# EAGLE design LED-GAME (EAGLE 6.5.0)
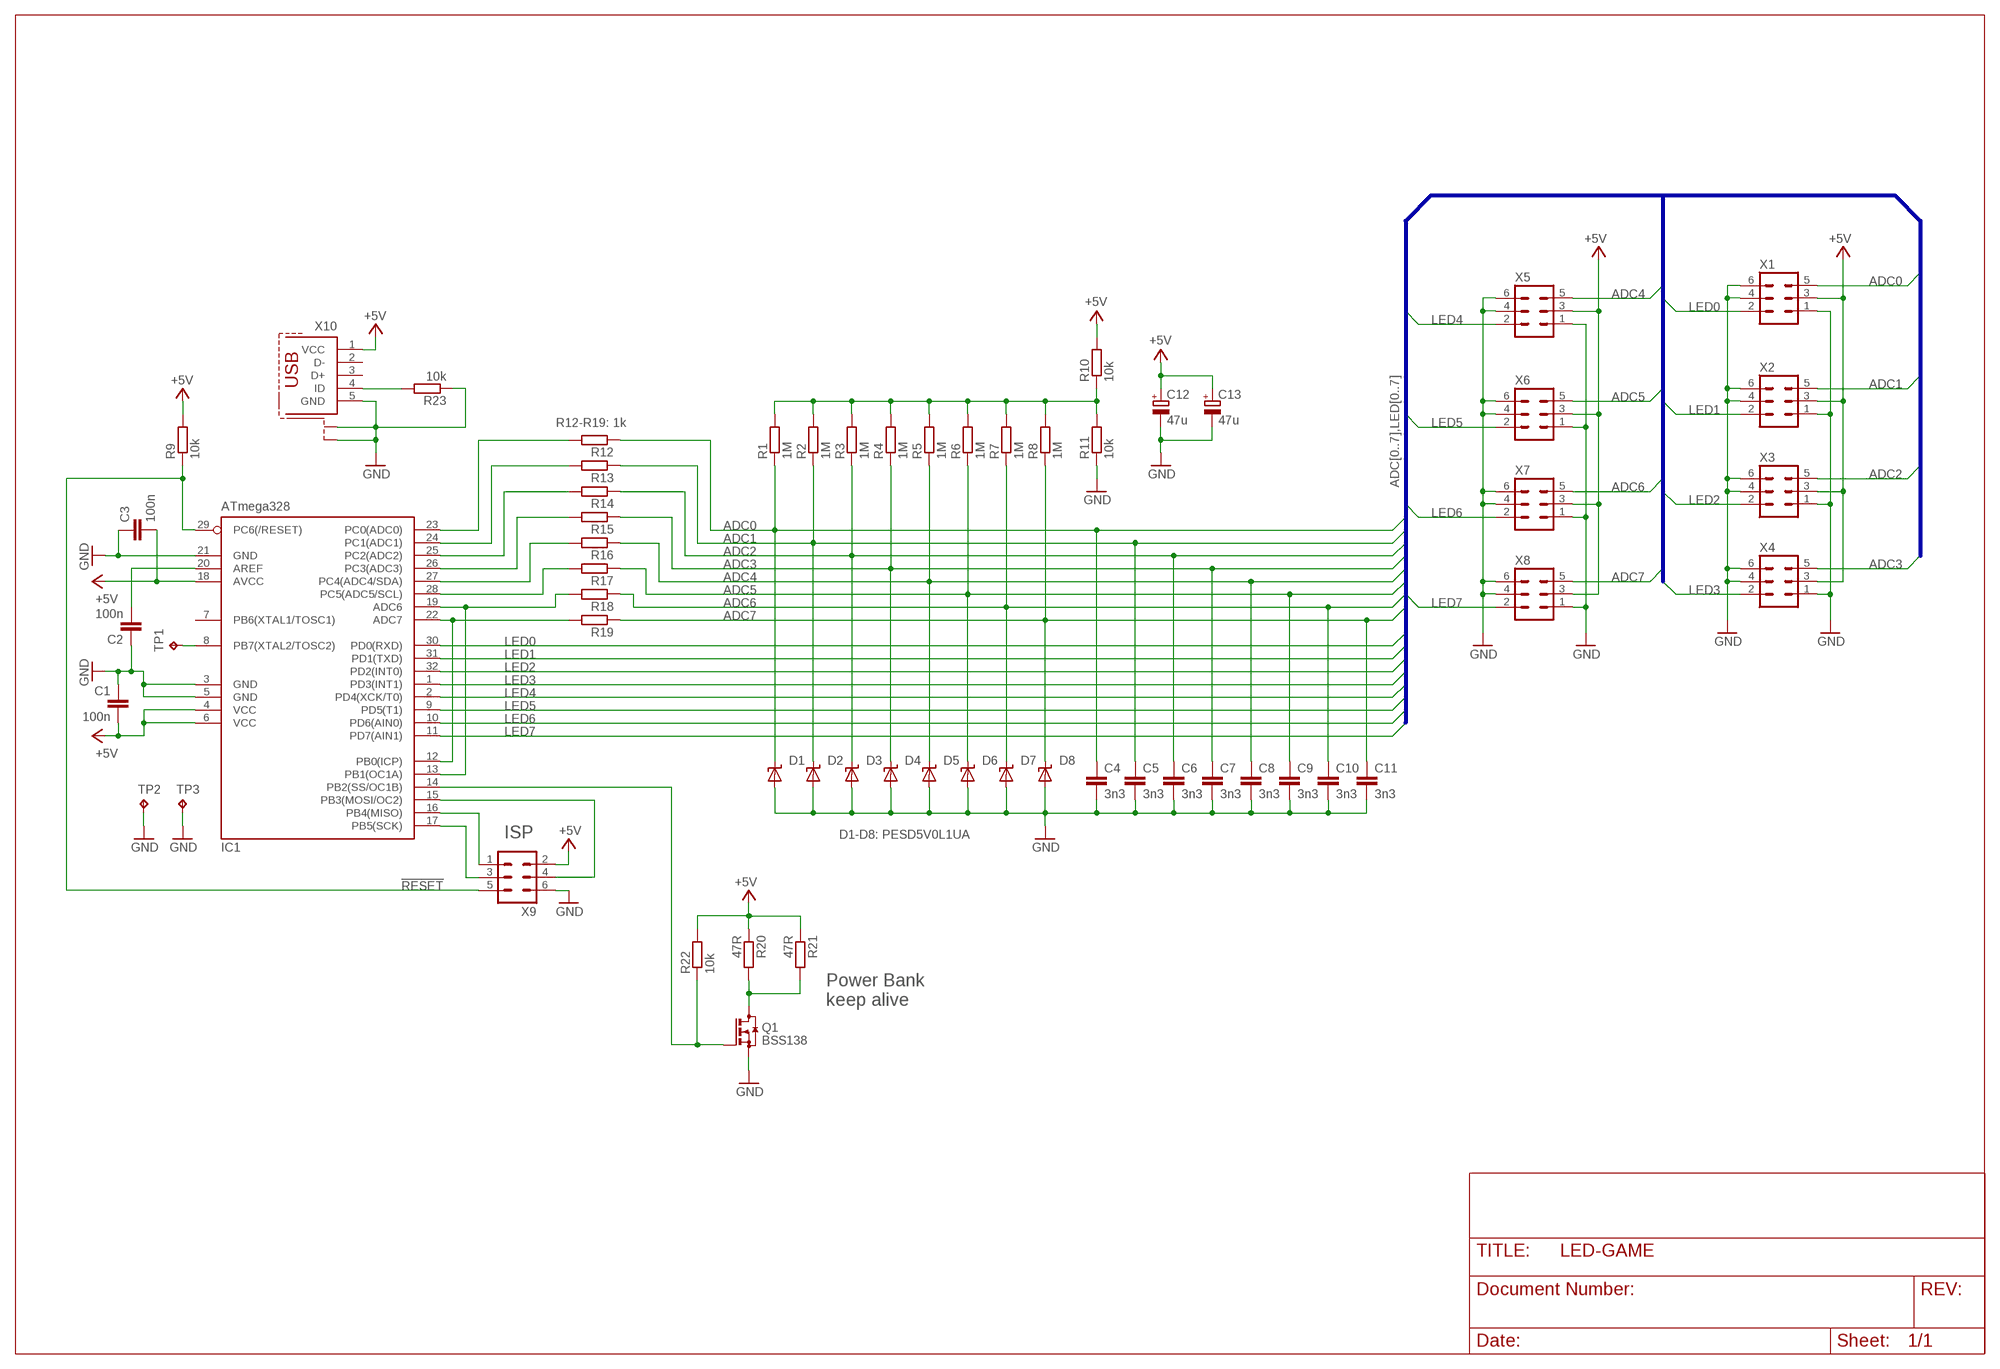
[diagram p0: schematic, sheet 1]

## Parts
C1  100n  C-EUC0603  [C0603]
C2  100n  C-EUC0603  [C0603]
C3  100n  C-EUC0603  [C0603]
C4  3n3  C-EUC0603K  [C0603K]
C5  3n3  C-EUC0603K  [C0603K]
C6  3n3  C-EUC0603K  [C0603K]
C7  3n3  C-EUC0603K  [C0603K]
C8  3n3  C-EUC0603K  [C0603K]
C9  3n3  C-EUC0603K  [C0603K]
C10  3n3  C-EUC0603K  [C0603K]
C11  3n3  C-EUC0603K  [C0603K]
C12  47u  CPOL-EUB/3528-21R  [B/3528-21R]
C13  47u  CPOL-EUB/3528-21R  [B/3528-21R]
D1  PESD5V  SUPPRESSOR_UNI  [SOD323-W]
D2  PESD5V  SUPPRESSOR_UNI  [SOD323-W]
D3  PESD5V  SUPPRESSOR_UNI  [SOD323-W]
D4  PESD5V  SUPPRESSOR_UNI  [SOD323-W]
D5  PESD5V  SUPPRESSOR_UNI  [SOD323-W]
D6  PESD5V  SUPPRESSOR_UNI  [SOD323-W]
D7  PESD5V  SUPPRESSOR_UNI  [SOD323-W]
D8  PESD5V  SUPPRESSOR_UNI  [SOD323-W]
IC1  ATmega328  MEGA8-AI  [TQFP32-08]
Q1  BSS138  BSS123  [SOT23]
R1  1M  R-EU_R0603  [R0603]
R2  1M  R-EU_R0603  [R0603]
R3  1M  R-EU_R0603  [R0603]
R4  1M  R-EU_R0603  [R0603]
R5  1M  R-EU_R0603  [R0603]
R6  1M  R-EU_R0603  [R0603]
R7  1M  R-EU_R0603  [R0603]
R8  1M  R-EU_R0603  [R0603]
R9  10k  R-EU_R0603  [R0603]
R10  10k  R-EU_R0603  [R0603]
R11  10k  R-EU_R0603  [R0603]
R12  1k  R-EU_R0603  [R0603]
R13  1k  R-EU_R0603  [R0603]
R14  1k  R-EU_R0603  [R0603]
R15  1k  R-EU_R0603  [R0603]
R16  1k  R-EU_R0603  [R0603]
R17  1k  R-EU_R0603  [R0603]
R18  1k  R-EU_R0603  [R0603]
R19  1k  R-EU_R0603  [R0603]
R20  47R  R-EU_R1206  [R1206]
R21  47R  R-EU_R1206  [R1206]
R22  10k  R-EU_R0603  [R0603]
R23  10k  R-EU_R0603  [R0603]
TP1  TPP1-08  [P1-08]
TP2  TPP1-08  [P1-08]
TP3  TPP1-08  [P1-08]
X1  ML6  [ML6]
X2  ML6  [ML6]
X3  ML6  [ML6]
X4  ML6  [ML6]
X5  ML6  [ML6]
X6  ML6  [ML6]
X7  ML6  [ML6]
X8  ML6  [ML6]
X9  ML6  [ML6]
X10  USBMICRO  [MOLEX_USB_MICRO_SD-47346-001]

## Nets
!RESET: IC1.29(PC6(/RESET)) R9.1 X9.5
+5V: C1.2 C3.2 C12.+ C13.+ IC1.4(VCC) IC1.6(VCC) IC1.18(AVCC) R9.2 R10.2 R20.1 R21.1 R22.2 X1.3 X2.3 X3.3 X4.3 X5.3 X6.3 X7.3 X8.3 X9.2 X10.1(VCC)
ADC0: C4.1 D1.C R1.1 R12.1 X1.5
ADC1: C5.1 D2.C R2.1 R13.1 X2.5
ADC2: C6.1 D3.C R3.1 R14.1 X3.5
ADC3: C7.1 D4.C R4.1 R15.1 X4.5
ADC4: C8.1 D5.C R5.1 R16.1 X5.5
ADC5: C9.1 D6.C R6.1 R17.1 X6.5
ADC6: C10.1 D7.C R7.1 R18.1 X7.5
ADC7: C11.1 D8.C R8.1 R19.1 X8.5
GND: C1.1 C2.1 C3.1 C4.2 C5.2 C6.2 C7.2 C8.2 C9.2 C10.2 C11.2 C12.- C13.- D1.A D2.A D3.A D4.A D5.A D6.A D7.A D8.A IC1.3(GND) IC1.5(GND) IC1.21(GND) Q1.2(S) R11.1 R23.1 TP2.TP TP3.TP X1.1 X1.4 X1.6 X2.1 X2.4 X2.6 X3.1 X3.4 X3.6 X4.1 X4.4 X4.6 X5.1 X5.4 X5.6 X6.1 X6.4 X6.6 X7.1 X7.4 X7.6 X8.1 X8.4 X8.6 X9.6 X10.5(GND) X10.M0(S1) X10.M1(S1) X10.M2(S1) X10.M3(S1) X10.M4(S2) X10.M5(S2) X10.M6(S2) X10.M7(S2) X10.M8(S1) X10.M9(S1) X10.M10(S2) X10.M11(S2)
LED0: IC1.30(PD0(RXD)) X1.2
LED1: IC1.31(PD1(TXD)) X2.2
LED2: IC1.32(PD2(INT0)) X3.2
LED3: IC1.1(PD3(INT1)) X4.2
LED4: IC1.2(PD4(XCK/T0)) X5.2
LED5: IC1.9(PD5(T1)) X6.2
LED6: IC1.10(PD6(AIN0)) X7.2
LED7: IC1.11(PD7(AIN1)) X8.2
N$1: C2.2 IC1.20(AREF)
N$2: IC1.8(PB7(XTAL2/TOSC2)) TP1.TP
N$3: IC1.23(PC0(ADC0)) R12.2
N$4: R1.2 R2.2 R3.2 R4.2 R5.2 R6.2 R7.2 R8.2 R10.1 R11.2
N$5: IC1.24(PC1(ADC1)) R13.2
N$6: IC1.16(PB4(MISO)) X9.1
N$7: IC1.17(PB5(SCK)) X9.3
N$8: IC1.26(PC3(ADC3)) R15.2
N$9: IC1.25(PC2(ADC2)) R14.2
N$10: IC1.27(PC4(ADC4/SDA)) R16.2
N$11: IC1.15(PB3(MOSI/OC2)) X9.4
N$12: IC1.28(PC5(ADC5/SCL)) R17.2
N$13: IC1.14(PB2(SS/OC1B)) Q1.1(G) R22.1
N$14: Q1.3(D) R20.2 R21.2
N$15: IC1.12(PB0(ICP)) IC1.22(ADC7) R19.2
N$16: IC1.13(PB1(OC1A)) IC1.19(ADC6) R18.2
N$17: R23.2 X10.4(ID)
Unconnected: IC1.7(PB6(XTAL1/TOSC1)) X10.2(D-) X10.3(D+)

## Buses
ADC[0..7],LED[0..7]

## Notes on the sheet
- R12-R19: 1k
- ISP | D1-D8: PESD5V0L1UA
- Power Bank
  keep alive

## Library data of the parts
C1-C11 = rcl:C-EU: CAPACITOR, European symbol
C12 C13 = rcl:CPOL-EU: POLARIZED CAPACITOR, European symbol
D1-D8 = Brunner:SUPPRESSOR_UNI
IC1 = atmel:MEGA8: MICROCONTROLLER 8 Kbytes FLASH, 1 kbytes SRAM, 512 bytes EEPROM, USART, 6-channel 10 bit ADC, 2-channel 8 bit ADC Pin compatible with Atmega48, ATMega88, ATMega168 Source: avr.lbr; MPN: ATMEGA8-16AU; OC_FARNELL: 9171371; OC_NEWARK: 73M8863
Q1 = transistor-small-signal:BSS123: N-CHANNEL MOS FET
R1-R23 = rcl:R-EU_: RESISTOR, European symbol
TP1-TP3 = testpad:TP: Test pad
X1-X9 = con-harting-ml:ML6: HARTING; OC_FARNELL: unknown; OC_NEWARK: unknown
X10 = Brunner:USB

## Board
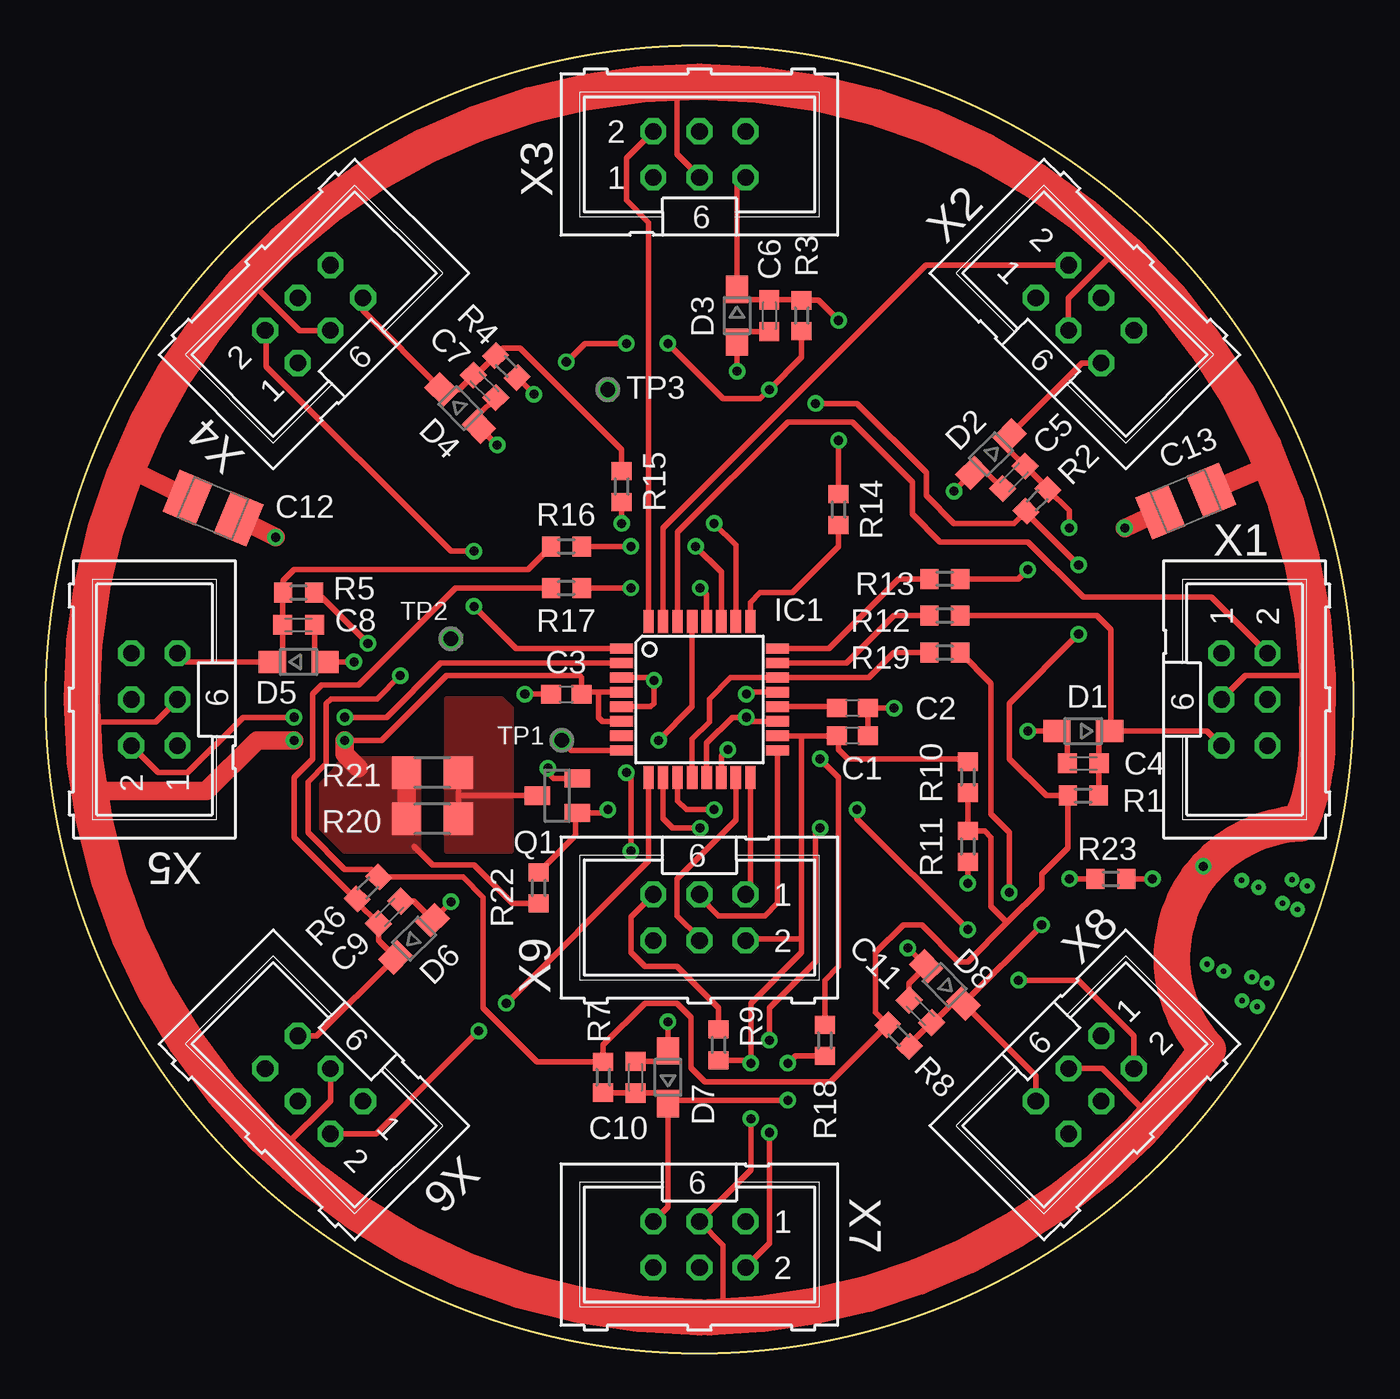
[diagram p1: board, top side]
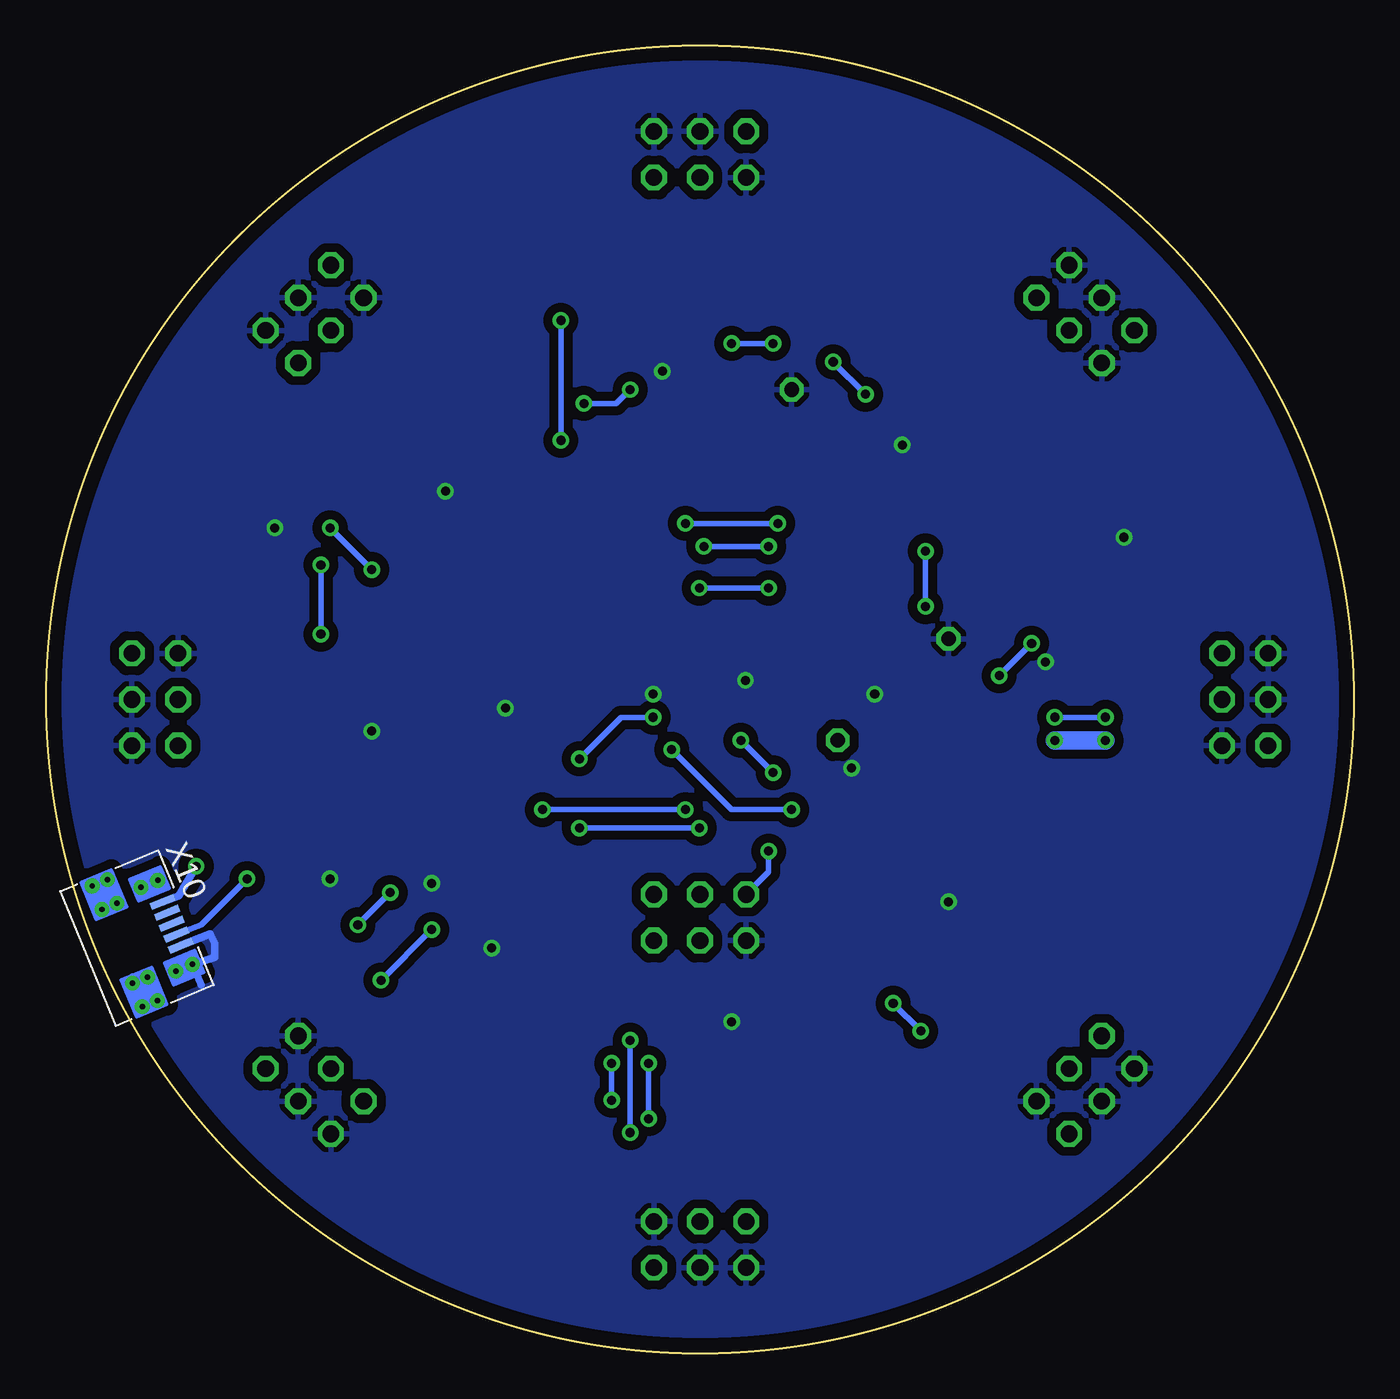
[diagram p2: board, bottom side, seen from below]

Size 72 x 72 mm. Coordinates in mm from the lower left corner, seen from the top.
Outline: circle at 36,36 radius 36
Copper layers (1*16): Top 0.035mm / dielectric 1.5mm / Bottom 0.035mm
Design rules "default *": minimum track width 0.3mm, minimum drill 0.5mm, track to track 0.3mm, track to pad 0.3mm, pad to pad 0.22mm, via to via 0.3mm, smd to smd 8mil, copper to edge 0.8mm, drill to drill 8mil, minimum pad ring 10mil, minimum via ring 8mil, stop-mask expansion 4mil, vias tented up to drill 0mil, thermal gap 0.3mm
bRestrict: 4 lines

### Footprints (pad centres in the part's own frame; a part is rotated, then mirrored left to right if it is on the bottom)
C0603 = smd 1.1 x 1: 1 -0.85,0; 2 0.85,0
C0603K = smd 1.05 x 1.08: 1 -0.875,0; 2 0.875,0
B/3528-21R = smd 1.95 x 2.5: + 1.525,0; - -1.525,0
SOD323-W = smd 1.5 x 1.2: A 1.45,0; C -1.45,0
TQFP32-08 = smd 1.27 x 0.559: 1 -4.293,2.8; 2 -4.293,2; 3 -4.293,1.2; 4 -4.293,0.4; 5 -4.293,-0.4; 6 -4.293,-1.2; 7 -4.293,-2; 8 -4.293,-2.8; 17 4.293,-2.8; 18 4.293,-2; 19 4.293,-1.2; 20 4.293,-0.4; 21 4.293,0.4; 22 4.293,1.2; 23 4.293,2; 24 4.293,2.8 | smd 0.559 x 1.27: 9 -2.8,-4.293; 10 -2,-4.293; 11 -1.2,-4.293; 12 -0.4,-4.293; 13 0.4,-4.293; 14 1.2,-4.293; 15 2,-4.293; 16 2.8,-4.293; 25 2.8,4.293; 26 2,4.293; 27 1.2,4.293; 28 0.4,4.293; 29 -0.4,4.293; 30 -1.2,4.293; 31 -2,4.293; 32 -2.8,4.293
SOT23 = smd 1 x 1.4: 1 -0.95,-1.1; 2 0.95,-1.1; 3 0,1.1
R0603 = smd 1 x 1.1: 1 -0.85,0; 2 0.85,0
R1206 = smd 1.6 x 1.803: 1 -1.422,0; 2 1.422,0
P1-08 = drill 0.8 octagon: TP 0,0
ML6 = drill 0.914 octagon: 1 -2.54,-1.27; 2 -2.54,1.27; 3 0,-1.27; 4 0,1.27; 5 2.54,-1.27; 6 2.54,1.27
MOLEX_USB_MICRO_SD-47346-001 = smd 0.4 x 1.4: 1 -1.3,2.85; 2 -0.65,2.85; 3 0,2.85; 4 0.65,2.85; 5 1.3,2.85 | drill 0.3: M0 -3.6,0.5; M1 -2.2,0.5; M2 -3.6,-0.4; M3 -2.2,-0.4; M4 2.2,0.5; M5 3.6,0.5; M6 2.2,-0.4; M7 3.6,-0.4; M8 -2.5,3.05; M9 -2.5,2.05; M10 2.5,3.05; M11 2.5,2.05

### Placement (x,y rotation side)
C1  44.42,34.01 180 top
C2  44.42,35.53 180 top
C3  28.67,36.29 0 top
C4  57.12,32.48 180 top
C5  53.31,48.23 225 top
C6  39.85,57.12 270 top
C7  24.17,53.24 315 top
C8  13.94,40.1 0 top
C9  18.95,24.28 45 top
C10  32.48,15.21 90 top
C11  48.16,18.84 135 top
C12  9.23,46.53 157.5 top
C13  62.77,46.92 22.5 top
D1  57.12,34.26 180 top
D2  52.04,49.5 225 top
D3  38.07,57.12 270 top
D4  22.83,52.04 315 top
D5  13.94,38.07 0 top
D6  20.29,22.83 45 top
D7  34.26,15.21 90 top
D8  49.5,20.29 135 top
IC1  36,36 0 top
Q1  28.16,30.7 90 top
R1  57.12,30.7 180 top
R2  54.58,46.96 225 top
R3  41.63,57.12 270 top
R4  25.37,54.33 315 top
R5  13.94,41.88 0 top
R6  17.75,25.62 45 top
R7  30.7,15.21 90 top
R8  46.96,17.5 135 top
R9  37.05,16.99 270 top
R10  50.77,31.72 90 top
R11  50.77,27.91 90 top
R12  49.5,40.61 180 top
R13  49.5,42.64 180 top
R14  43.66,46.45 270 top
R15  31.72,47.72 270 top
R16  28.67,44.42 0 top
R17  28.67,42.13 0 top
R18  42.9,17.24 90 top
R19  49.5,38.58 180 top
R20  21.31,29.43 0 top
R21  21.31,31.97 0 top
R22  27.15,25.62 270 top
R23  58.64,26.13 0 top
TP1  28.42,33.75 0 top
TP2  22.32,39.34 0 top
TP3  30.96,53.06 0 top
X1  66,36 270 top
X2  57.21,57.21 315 top
X3  36,66 0 top
X4  14.79,57.21 45 top
X5  6,36 90 top
X6  14.79,14.79 135 top
X7  36,6 180 top
X8  57.21,14.79 225 top
X9  36,24 180 top
X10  67.71,22.57 292.5 bottom

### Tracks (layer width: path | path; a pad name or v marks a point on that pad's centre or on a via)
!RESET  (via drill 0.5)
  Top 0.305: IC1.29 35.6,35.6 v33.75,33.75 | v31.97,31.97 32.23,31.72 v32.23,27.66 | R9.1 37.05,19.02 34.77,21.31 32.99,21.31 32.23,22.07 32.23,24.04 X9.5
  Bottom 0.305: X9.5 32.23,26.5 v32.23,27.66 | v31.97,31.97 v33.75,33.75
+5V  (via drill 0.5)
  Top 0.305: X3.3 36,64.78 34.77,66.01 34.77,70 36,70 | IC1.18 41.63,34 | 41.63,34 C1.2 43.66,34.01 43.66,33.24 44.17,32.74 50.6,32.74 R10.2 | 2.23,34.77 6.07,34.77 7.27,35.97 X5.3 7.31,36.04 | X8.3 58.17,15.68 60.68,13.18 | 60.68,13.18 60.85,13 61,13 | X1.3 66.04,37.31 69.69,37.31 | X2.3 56.31,58.09 58.9,60.68 | 58.9,60.68 59,60.78 59,61 | 41.63,22.83 41.63,22.07 38.83,19.27 38.83,16.14 | 41.63,22.83 41.63,34 | v38.83,12.92 38.83,10.1 X7.3 37.31,5.96 37.31,2.31 37,2 36.54,2 36,2 | 2.23,34.77 arc-90 2,35 2,36 2.51,42.13 3.78,47.21 4.57,48.73 7.84,55.09 11.3,58.54 11.3,59 | 11.3,59 11,59 | 69.69,37.31 arc-90 70,37 70,34 69.82,30.7 | 2.58,30.84 3.27,26.89 5.81,20.29 9.11,14.96 12.67,11.4 13.18,11.4 15.68,13.91 X6.3 | 2.58,30.84 2.51,31.21 2.23,34.77 | X4.3 13.98,56.31 11.3,59 | 58.9,60.68 63.22,56.36 66.77,50.52 67.37,48.86 68.8,44.93 69.82,39.09 69.69,37.31 | 60.68,13.18 61.44,13.18 | X9.2 38.73,22.73 38.83,22.83 41.63,22.83 | IC1.4 30.45,36.4 | 30.45,36.4 29.63,36.4 C3.2 29.52,37.22 29.43,37.31 22.07,37.31 18.51,33.75 v16.48,33.75 | IC1.6 30.67,34.8 30.45,35.02 30.45,36.4 | 2.7,30.96 2.58,30.84 | 20.46,28.86 R20.1 | 69.06,29.18 65.26,27.84 v63.73,26.82 | R22.2 25.71,24.77 23.59,26.89 21.31,26.89 20.29,27.91 | R9.2 38.83,16.14 | 38.83,16.14 v38.83,15.97
  Top 0.406: 63.98,16.73 61.44,13.18
  Top 1.016: v13.69,33.75 11.65,33.75 8.86,30.96 2.7,30.96 | R20.1 R21.1 | v16.48,33.75 16.48,32.99 17.24,32.23 | C12.+ 4.57,48.73 | C13.+ 67.37,48.86
  Top 2: 36,2 arc-90 2,36 arc-90 36,70 arc-93 70,34 arc-25 69.06,29.18 arc130 63.98,16.73 arc-54 36.54,2
  Bottom 0.305: v38.83,15.97 v38.83,12.92
  Bottom 0.406: X10.1 64.7,25.2 v63.73,26.82
  Bottom 1.016: v16.48,33.75 v13.69,33.75
  pour Top (no thermals): 20.54,32.74 16.48,32.74 15.21,31.47 15.21,28.93 16.48,27.66 20.54,27.66
ADC0
  Top 0.305: X1.5 63.93,34.26 D1.C 58.64,34.33 58.64,34.77 | 58.64,34.77 58.64,39.85 57.88,40.61 R12.1 | 58.64,34.77 58,34.12 C4.1 58,30.73 R1.1
ADC1  (via drill 0.5)
  Top 0.305: X2.5 57.06,54.52 D2.C 53.06,49.71 | 53.06,49.68 53.06,49.71 | 53.06,49.71 C5.1 55.18,47.6 R2.1 56.36,46.38 v56.36,45.44 | R13.1 53.56,42.64 v54.07,43.15
  Bottom 0.305: v54.07,43.15 v56.36,45.44
ADC2  (via drill 0.5)
  Top 0.305: X3.5 38.07,64.26 D3.C arc90 38.65,58 C6.1 41.6,58 R3.1 42.55,57.97 v43.66,56.87 | R14.1 v43.66,50.26
  Bottom 0.305: v43.66,50.26 v43.66,56.87
ADC3
  Top 0.305: X4.5 17.48,57.39 D4.C 22.77,53.06 C7.1 23.7,53.85 R4.1 25.18,55.34 26.13,55.34 31.72,49.75 R15.1
ADC4
  Top 0.305: X5.5 7.74,38.07 D5.C 13.07,38.65 C8.1 13.07,41.85 R5.1 13.09,42.55 13.69,43.15 26.55,43.15 R16.1
ADC5
  Top 0.305: X6.5 14.94,17.48 D6.C 18.33,22.74 C9.1 17.15,24.84 R6.1 17.08,25.02 13.69,28.42 13.69,31.72 14.7,32.74 14.7,36.29 15.21,36.8 17.24,36.8 22.58,42.13 R17.1
ADC6  (via drill 0.5)
  Top 0.305: D7.C 34.26,8.07 X7.5 | D7.C 33.69,14.34 C10.1 30.73,14.34 R7.1 | D7.C 34.44,13.94 v40.86,13.94 | v40.86,15.97 41.28,16.39 R18.1
  Bottom 0.305: v40.86,13.94 v40.86,15.97
ADC7  (via drill 0.5)
  Top 0.305: D8.C 54.52,15.27 X8.5 | D8.C 49.93,19.27 48.89,18.22 C11.1 47.56,17.01 R8.1 | v53.06,25.37 53.06,28.67 52.04,29.69 52.04,36.89 R19.1 | v54.83,23.59 54.83,23.57 D8.C
  Bottom 0.305: v53.06,25.37 v54.83,23.59
GND  (via drill 0.5)
  Top 0.305: IC1.3 33.35,37.2 v33.5,37.05 33.5,35.78 33.31,35.6 IC1.5 | C3.1 v26.39,36.29 | v46.71,35.53 C2.1 C1.1 | IC1.21 38.69,36.4 v38.58,36.29 | v16.99,38.07 D5.A 14.82,38.65 C8.2 | v34.26,18.26 D7.A 33.69,16.09 C10.2 | v47.47,22.32 D8.A 47.54,20.38 C11.2 | v47.47,22.32 | v54.07,34.26 D1.A 56.25,34.26 C4.2 | v50.01,47.47 D2.A 51.83,48.48 C5.2 | v38.07,54.07 D3.A 38.65,56.25 C6.2 | v24.86,50.01 D4.A 23.85,51.68 C7.2 | v24.86,50.01 | v22.32,24.86 D6.A 20.27,24.9 C9.2 | R11.1 v50.77,25.88 | R23.1 v56.37,26.13 | Q1.2 27.98,31.65 27.66,31.97 v27.66,32.23
  Top 1.016: C12.- v12.67,44.93 | C13.- v59.41,45.44
  Bottom 0.406: X10.M1 68.92,24.79 X10.M3 | X10.M4 67.23,20.72 X10.M6 | X10.5 62.96,23.08 62.71,22.58 62.71,21.81 X10.M10 63.47,20.29
  pour Bottom (isolate 0.5): -1.3,73.63 73.63,73.63 73.63,-1.3 -1.3,-1.3
LED0
  Top 0.305: IC1.30 34.8,45.21 40.86,51.28 44.42,51.28 47.72,47.98 47.72,46.2 49.25,44.67 54.07,44.67 57.12,41.63 64.18,41.63 X1.2
LED1
  Top 0.305: IC1.31 34,45.43 48.48,59.91 X2.2
LED2
  Top 0.305: IC1.32 33.2,62.24 31.97,63.47 31.97,65.78 X3.2
LED3  (via drill 0.5)
  Top 0.305: IC1.1 25.91,38.8 v23.59,41.12 | v23.59,44.17 22.32,44.17 12.16,54.33 12.16,56.25 X4.2
  Bottom 0.305: v23.59,41.12 v23.59,44.17
LED4  (via drill 0.5)
  Top 0.305: X5.2 6.22,31.97 7.84,31.97 10.89,35.02 v13.69,35.02 | v16.48,35.02 18.77,35.02 21.74,38 IC1.2
  Bottom 0.305: v13.69,35.02 v16.48,35.02
LED5  (via drill 0.5)
  Top 0.305: IC1.9 33.2,27.1 v25.37,19.27 | X6.2 18.19,12.09 v23.85,17.75
  Bottom 0.305: v23.85,17.75 v25.37,19.27
LED6  (via drill 0.5)
  Top 0.305: X7.2 38.54,4.76 39.85,6.07 v39.85,12.16 | v39.85,17.24 39.85,19.02 42.39,21.56 42.39,28.67 v42.64,28.93 | IC1.10 34,29.44 34.51,28.93 v36.04,28.93
  Bottom 0.305: v39.85,12.16 v39.85,17.24 | v42.64,28.93 v36.04,28.93
LED7  (via drill 0.5)
  Top 0.305: IC1.11 34.8,30.42 35.28,29.94 v36.8,29.94 | v44.67,29.94 44.67,29.43 v50.77,23.34 | v53.56,20.54 56.87,20.54 59.91,17.5 59.91,15.69 X8.2
  Bottom 0.305: v36.8,29.94 v44.67,29.94 | v50.77,23.34 v53.56,20.54
N$1
  Top 0.305: IC1.20 43.5,35.6 C2.2
N$2
  Top 0.305: IC1.8 28.97,33.2 TP1.TP
N$3
  Top 0.305: IC1.23 44.1,38 46.71,40.61 R12.2
N$4  (via drill 0.5)
  Top 0.305: R4.2 26.64,53.06 v26.89,52.8 | v28.67,54.58 29.69,55.6 v31.97,55.6 | v34.26,55.6 37.31,52.55 39.34,52.55 v39.85,53.06 41.63,54.83 R3.2 | 52.93,23.72 54.83,25.62 54.83,26.39 56.27,27.82 R1.2 55.09,30.7 53.06,32.74 53.06,35.78 v56.87,39.59 | v19.53,37.31 18.26,36.04 15.72,36.04 15.46,35.78 15.46,32.48 14.45,31.47 14.45,28.67 16.48,26.64 17.94,26.64 R6.2 | R10.1 R11.2 51.7,28.76 52.04,28.42 52.04,24.61 52.93,23.72 | v42.39,52.29 44.67,52.29 48.48,48.48 48.48,47.21 50.01,45.69 53.31,45.69 R2.2 53.98,46.29 v56.87,43.4 | 52.93,23.72 50.77,21.56 50.26,21.56 48.23,23.59 47.21,23.59 45.69,22.07 45.69,18.77 R8.2 43.22,14.96 36.29,14.96 35.53,15.72 35.53,18.51 34.77,19.27 32.99,19.27 30.7,16.99 R7.2 27.06,16.06 24.1,19.02 24.1,25.12 22.99,26.23 R6.2 | R6.2 18.26,26.32 18.07,26.32 | R5.2 14.96,41.88 v17.75,39.09
  Bottom 0.305: v26.89,52.8 v28.67,54.58 | v31.97,55.6 v34.26,55.6 | v39.85,53.06 40.61,52.29 v42.39,52.29 | v56.87,43.4 v56.87,39.59 | v19.53,37.31 v17.75,39.09
N$5
  Top 0.305: IC1.24 43.12,38.8 46.96,42.64 R13.2
N$6
  Top 0.305: IC1.16 38.8,25.53 X9.1
N$7
  Top 0.305: IC1.17 40.29,24.8 39.59,24.1 37.05,24.1 36,25.15 X9.3
N$8  (via drill 0.5)
  Top 0.305: IC1.26 38,44.49 v36.8,45.69 | v31.72,45.69 R15.2
  Bottom 0.305: v36.8,45.69 v31.72,45.69
N$9
  Top 0.305: IC1.25 38.8,41.34 39.34,41.88 41.12,41.88 43.66,44.42 R14.2
N$10  (via drill 0.5)
  Top 0.305: IC1.27 37.2,43 v35.78,44.42 | v32.23,44.42 R16.2
  Bottom 0.305: v35.78,44.42 v32.23,44.42
N$11
  Top 0.305: IC1.15 38,29.36 34.77,26.13 34.77,24.1 36,22.87 X9.4
N$12  (via drill 0.5)
  Top 0.305: IC1.28 36.4,41.77 v36.04,42.13 | v32.23,42.13 R17.2
  Bottom 0.305: v36.04,42.13 v32.23,42.13
N$13  (via drill 0.5)
  Top 0.305: IC1.14 37.2,32.88 v37.56,33.24 | v30.96,29.94 30.77,29.75 Q1.1 29.18,29.67 29.18,28.51 R22.1
  Bottom 0.305: v30.96,29.94 34.26,29.94 v37.56,33.24
N$14
  Top 0.305: R20.2 22.73,30.7 | 22.73,30.7 R21.2 | Q1.3 22.73,30.7
  pour Top (no thermals): 22.07,27.66 22.07,36.04 25.12,36.04 25.62,35.53 25.62,27.66
N$15
  Top 0.305: R19.2 46.71,38.58 45.33,37.2 IC1.22 37.71,37.2 36.55,36.04 36.55,34.77 35.6,33.82 IC1.12
N$16  (via drill 0.5)
  Top 0.305: R18.2 42.9,20.54 43.66,21.31 43.66,31.72 v42.64,32.74 | IC1.19 38.8,34.8 v38.58,35.02 37.82,35.02 36.4,33.61 IC1.13
  Bottom 0.305: v42.64,32.74 40.36,35.02 v38.58,35.02
N$17  (via drill 0.5)
  Top 0.305: R23.2 v60.93,26.13
  Bottom 0.305: X10.4 63.47,23.59 v60.93,26.13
